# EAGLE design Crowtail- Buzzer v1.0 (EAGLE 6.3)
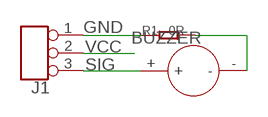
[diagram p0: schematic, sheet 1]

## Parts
BUZZER  BUZZER-YMD12065  [2P-7.6-D12X6.5H]
J1  TINKER_3P_DIP  [3P_2.0_DIP]
R1  0R  R-0603  [R0603]

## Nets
GND: J1.1 R1.1
N$1: BUZZER.- R1.2
SIG: BUZZER.+ J1.3
VCC: J1.2

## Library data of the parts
BUZZER = template:BUZZER-YMD12065
J1 = Connector:TINKER_3P_DIP
R1 = Discrete:R*

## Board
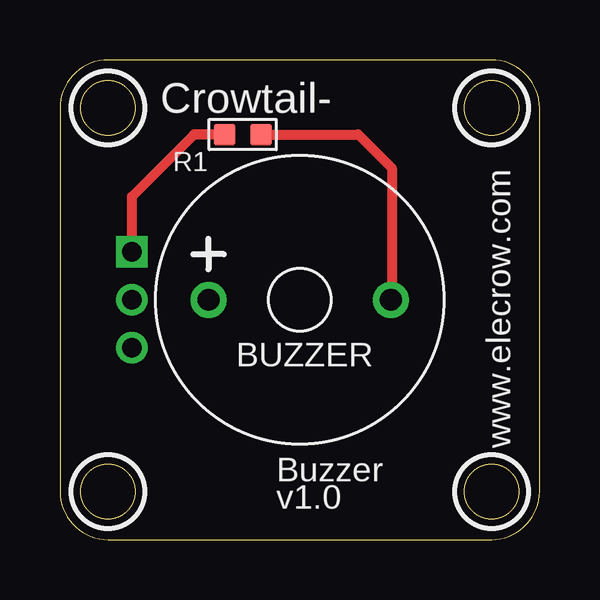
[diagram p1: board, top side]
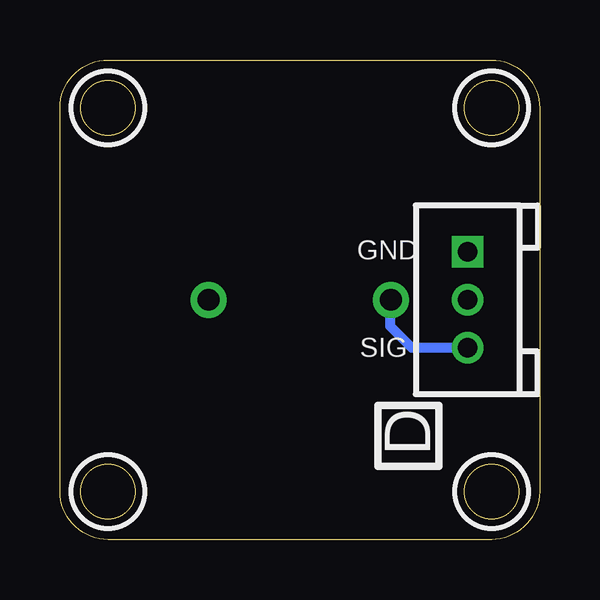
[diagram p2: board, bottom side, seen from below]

Size 20 x 20 mm. Coordinates in mm from the lower left corner, seen from the top.
Outline: 2,0 18,0 arc90 20,2 20,18 arc90 18,20 2,20 arc90 0,18 0,2 arc90 2,0
Outline: circle at 2,18 radius 1.14
Outline: circle at 2,2 radius 1.14
Outline: circle at 18,18 radius 1.14
Outline: circle at 18,2 radius 1.14
Copper layers (1*16): Top 0.035mm / dielectric 1.5mm / Bottom 0.035mm
Design rules "default": minimum track width 10mil, minimum drill 24mil, track to track 8mil, track to pad 8mil, pad to pad 8mil, via to via 8mil, smd to smd 8mil, copper to edge 40mil, drill to drill 8mil, minimum pad ring 10mil, minimum via ring 8mil, stop-mask expansion 4mil, vias tented up to drill 0mil, thermal gap 10mil
tRestrict: area 0.5,16.5 to 3.5,19.5; area 0.5,0.5 to 3.5,3.5; area 16.5,16.5 to 19.5,19.5; area 16.5,0.5 to 19.5,3.5
bRestrict: area 0.5,16.5 to 3.5,19.5; area 0.5,0.5 to 3.5,3.5; area 16.5,16.5 to 19.5,19.5; area 16.5,0.5 to 19.5,3.5

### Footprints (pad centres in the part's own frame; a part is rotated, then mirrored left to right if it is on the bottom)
2P-7.6-D12X6.5H = drill 0.9 pad 1.5: + -3.8,0; - 3.8,0
3P_2.0_DIP = drill 0.8 pad 1.27 square: 1 -2,0 | drill 0.8 pad 1.27: 2 0,0; 3 2,0
R0603 = smd 0.889 x 0.889: 1 -0.762,0; 2 0.762,0

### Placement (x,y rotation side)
BUZZER  10,10 0 top
J1  3,10 270 bottom
R1  7.62,16.89 0 top

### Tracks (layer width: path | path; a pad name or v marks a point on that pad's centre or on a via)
GND
  Top 0.406: J1.1 3,14.3 5.59,16.89 R1.1
N$1
  Top 0.406: BUZZER.- 13.84,10.04 13.84,15.49 12.45,16.89 R1.2
SIG
  Bottom 0.406: J1.3 5.33,8 6.22,8.89 6.22,9.98 BUZZER.+

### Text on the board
tPlace: Crowtail- | www.elecrow.com | Buzzer | v1.0
bPlace: GND | SIG | D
